(* Logix 5000 DataType export CM1T_Controlword; software revision 20.00 *)

TYPE CM1T_Controlword :
STRUCT
   Start : BOOL;   // Start a motion or set a new setpoint
   Halt : BOOL;   // Halt the current motion
   Relative_Move : BOOL;   // Execute the position profile as a relative move
   Speed_Control : BOOL;   // Execute the profile as speed control only
   Disable : BOOL;   // Disable the drive (zero torque)
   Reset_Error : BOOL;   // Reset any existing errors with rising edge
   Set_to_Zero : BOOL;   // Set the current position to 0
   Home : BOOL;   // Execute a home search
END_STRUCT
END_TYPE
